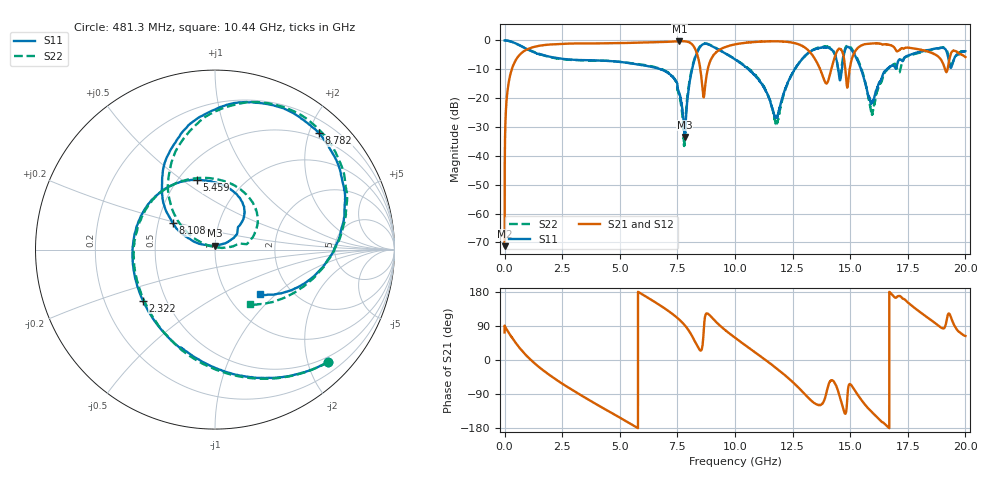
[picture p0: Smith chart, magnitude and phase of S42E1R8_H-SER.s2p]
! Created Wed Nov 25 21:36:40 2020
# khz S ma R 50
! 2 Port Network Data from SP1.SP block
! freq  magS11  angS11  magS21  angS21  magS12  angS12  magS22  angS22
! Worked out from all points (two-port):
!   20001 points, 300 kHz to 20 GHz, reference 50 ohm
!   highest |S21| = -0.25 dB at 7.586 GHz (marker M1); lowest = -71.3 dB at 300 kHz (marker M2)
!   |S21| within 3 dB of the highest: 939.6 MHz to 8.288 GHz (7.348 GHz wide, 159 % of centre); 9.327 GHz to 13.16 GHz (3.832 GHz wide, 34.1 % of centre)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
!   lowest |S11| = -33.5 dB at 7.817 GHz (marker M3), VSWR 1.04, Z = 49.8 + j2.1 ohm
!   |S11| at or under -10 dB: 6.78 GHz to 8.137 GHz (1.357 GHz wide, 18.2 % of centre); 10.58 GHz to 12.59 GHz (2.013 GHz wide, 17.4 % of centre); 15.47 GHz to 16.59 GHz (1.117 GHz wide, 6.97 % of centre)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
!   |S22| runs from -37.1 to 0.0 dB; largest |S21 - S12| = 0.019
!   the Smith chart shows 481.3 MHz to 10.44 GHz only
!   S11 on the Smith chart (normalised r, x): 481.3 MHz: 0.40, -2.36; 2.322 GHz: 0.37, -0.28; 5.459 GHz: 0.61, +0.57; 8.108 GHz: 0.60, +0.19; 8.782 GHz: 0.40, +2.17; 10.44 GHz: 1.40, -0.80
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300  0.9997 -0.2  0.0002719 72.7  0.0003016 93.3  0.9984 -0.3
129300  0.9894 -12.6  0.1378 77.0  0.1384 77.0  0.9895 -12.6
481300  0.8879 -45.0  0.4545 45.3  0.4559 45.4  0.8882 -44.8
2322300  0.4915 -144.7  0.8684 -55.3  0.869 -55.2  0.4842 -145.7
3334300  0.4577 173.9  0.8873 -93.6  0.8867 -93.7  0.4527 178.4
5459300  0.4022 104.7  0.9086 -168.1  0.9094 -168.2  0.4049 99.5
6667300  0.3264 67.2  0.9367 147.3  0.9348 147.2  0.3325 49.9
7586300  0.1205 32.0  0.9718 106.4  0.9689 106.5  0.1098 10.9
7817300  0.02114 95.0  0.9659 91.8  0.966 92.0  0.02111 126.4
8108300  0.2787 147.6  0.8771 66.2  0.8779 66.1  0.2973 139.3
8782300  0.8709 48.3  0.271 123.2  0.2719 123.3  0.881 45.7
1.00003e7  0.4706 -29.3  0.8556 58.8  0.8555 59.1  0.4733 -34.1
1.04363e7  0.3521 -45.0  0.9084 39.3  0.9085 39.3  0.3609 -57.4
1.18013e7  0.04591 -7.2  0.9672 -21.9  0.9675 -21.9  0.03431 147.3
1.33343e7  0.6634 -24.0  0.5732 -108.5  0.5785 -108.5  0.6708 -34.0
1.39713e7  0.7542 -79.4  0.1806 -85.6  0.1795 -86.6  0.7815 -85.6
1.45573e7  0.2041 -102.3  0.7138 -98.7  0.7151 -98.7  0.2474 -92.9
1.50003e7  0.733 -130.1  0.3613 -63.8  0.359 -63.6  0.776 -129.6
1.59423e7  0.08397 -127.3  0.8881 -137.4  0.8902 -137.2  0.05223 -132.6
1.66673e7  0.3348 -93.8  0.8438 -178.2  0.8327 -178.3  0.3311 -97.5
1.87683e7  0.7292 -176.8  0.5453 93.5  0.5462 93.5  0.7237 178.3
2e7  0.6473 152.6  0.5159 63.4  0.5178 64.5  0.668 136.2
